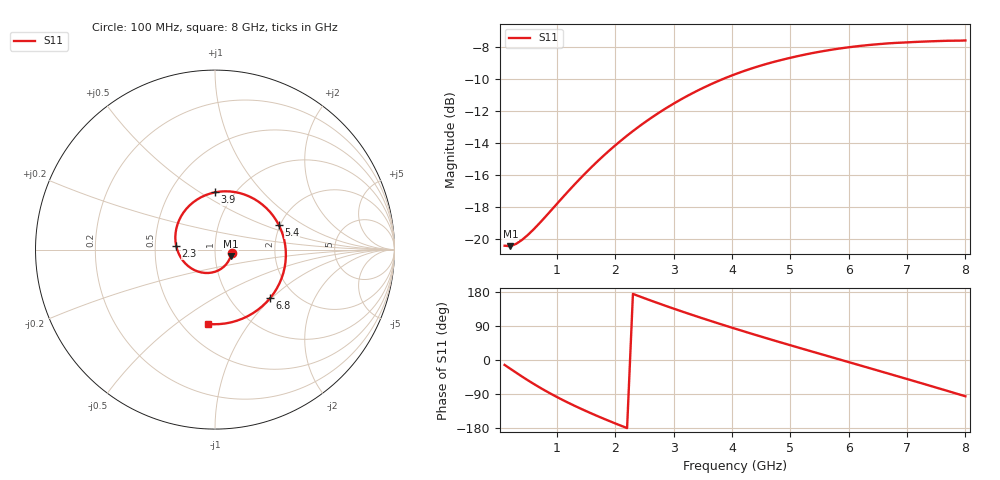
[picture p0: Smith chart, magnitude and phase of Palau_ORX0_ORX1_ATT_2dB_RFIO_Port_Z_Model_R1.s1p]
! Created Fri Oct  9 14:28:54 2020
! Palau ORX0/ORX1 RFIO Port Impedance Model.
! Attenuation  : 2 dB.
! Revision		: R1.
! Impedance Mode 	: Balanced Differential-Mode.
! Impedance Format 	: Series Equivalent Differential Impedance (SEDZ).
# hz S ma R 100
! 1 Port Network Data from SP1.SP block
! freq  magS11  angS11
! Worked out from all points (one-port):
!   80 points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, 100 MHz to 8 GHz, reference 100 ohm
!   lowest |S11| = -20.4 dB at 200 MHz (marker M1), VSWR 1.21, Z = 119 - j9.05 ohm
!   |S11| at or under -10 dB: start of sweep to 3.85 GHz
!   S11 on the Smith chart (normalised r, x): 100 MHz: 1.20, -0.05; 2.3 GHz: 0.64, +0.03; 3.9 GHz: 0.82, +0.58; 5.4 GHz: 1.97, +0.63; 6.8 GHz: 1.51, -0.98; 8 GHz: 0.66, -0.66
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1e8  0.09554 -13.0
2e8  0.09524 -23.3
4e8  0.09968 -43.8
7e8  0.1124 -72.4
1.1e9  0.1354 -105.8
1.3e9  0.1483 -120.8
1.6e9  0.1686 -141.8
1.8e9  0.1825 -155.0
2.1e9  0.2035 -173.7
2.3e9  0.2174 174.4
2.7e9  0.2449 151.7
3.1e9  0.2714 130.2
3.5e9  0.2962 109.7
3.9e9  0.3189 90.0
4.1e9  0.3294 80.4
4.3e9  0.3391 71.0
4.6e9  0.3524 57.1
4.8e9  0.3604 47.9
5.1e9  0.3714 34.4
5.4e9  0.3811 21.0
5.8e9  0.3921 3.3
6.1e9  0.3987 -10.0
6.4e9  0.404 -23.4
6.8e9  0.4092 -41.2
7.1e9  0.4118 -54.7
7.4e9  0.4139 -68.3
7.6e9  0.4151 -77.4
8e9  0.4165 -95.7
